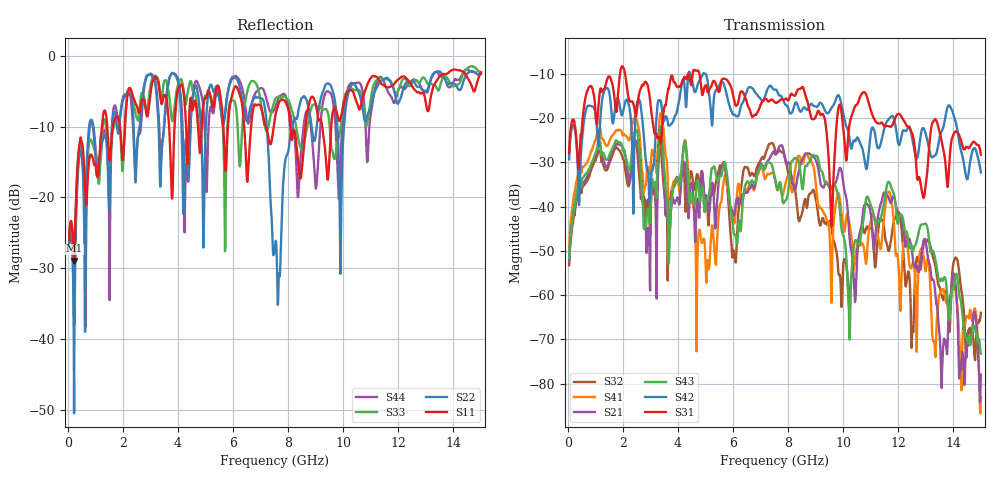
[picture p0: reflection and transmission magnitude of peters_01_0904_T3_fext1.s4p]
# MHZ S RI R 50.00
! FREQ  S11  S12  S13  S14
!  S21  S22  S23  S24
!  S31  S32  S33  S34
!  S41  S42  S43  S44
!  REAL  IMAG  REAL  IMAG  REAL  IMAG  REAL  IMAG
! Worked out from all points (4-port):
!   1496 points, 50 MHz to 15 GHz, reference 50 ohm
!   strongest paths, dB at 50 MHz, 3.79 GHz, 7.53 GHz, 11.27 GHz, 15 GHz:
!     S31: -27.9, -10.4, -16.4, -21.2, -28.2
!     S42: -29.3, -21.1, -13.5, -26.8, -32.2
!     S43: -51.6, -37.7, -33.8, -43.2, -73.2
!     S21: -52.4, -38.6, -28.1, -42.0, -78.0
!     S41: -49.1, -36.9, -34.1, -46.8, -83.2
!     S32: -53.3, -35.6, -27.2, -45.6, -64.0
!   lowest |S11| = -29.0 dB at 240 MHz (marker M1), VSWR 1.07, Z = 53.6 + j0.667 ohm
!   |S11| at or under -10 dB: start of sweep to 1.24 GHz; 8.078 GHz to 8.632 GHz (554.2 MHz wide, 6.63 % of centre); 9.237 GHz to 9.566 GHz (328.7 MHz wide, 3.5 % of centre)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
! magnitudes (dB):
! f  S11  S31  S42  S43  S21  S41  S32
! 50 MHz  -26.0  -27.9  -29.3  -51.6  -52.4  -49.1  -53.3
! 240 MHz  -29.0  -20.7  -22.0  -39.3  -40.7  -36.7  -41.2
! 5.08 GHz  -5.1  -14.2  -11.7  -38.1  -38.9  -52.2  -41.4
! 8.77 GHz  -6.6  -18.1  -17.3  -30.0  -28.0  -29.3  -37.2
! 10.22 GHz  -4.9  -21.8  -24.1  -66.6  -46.2  -43.4  -62.0
! 11.66 GHz  -4.5  -21.8  -20.2  -34.4  -38.2  -36.6  -50.0
! 15 GHz  -2.3  -28.2  -32.2  -73.2  -78.0  -83.2  -64.0
